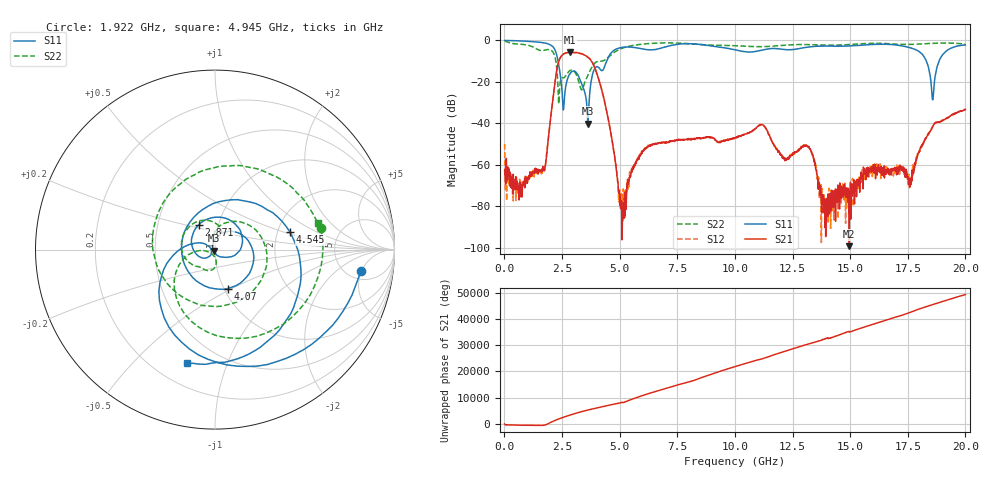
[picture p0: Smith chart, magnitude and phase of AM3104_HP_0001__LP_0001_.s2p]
!Created with skrf (http://scikit-rf.org).
# Hz S RI R 50.0
!freq ReS11 ImS11 ReS21 ImS21 ReS12 ImS12 ReS22 ImS22
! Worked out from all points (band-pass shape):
!   1601 points, 10 MHz to 20 GHz, reference 50 ohm
!   highest |S21| = -5.71 dB at 2.834 GHz (marker M1); lowest = -99.2 dB at 14.97 GHz (marker M2)
!   |S21| within 3 dB of the highest: 2.406 GHz to 3.696 GHz (1.29 GHz wide, 42.3 % of centre)
!   lowest |S11| = -40.1 dB at 3.621 GHz (marker M3), VSWR 1.02, Z = 49.2 - j0.591 ohm
!   |S11| at or under -10 dB: 2.33 GHz to 4.433 GHz (2.103 GHz wide, 62.2 % of centre); 18.31 GHz to 18.86 GHz (548.1 MHz wide, 2.95 % of centre)
!   |S22| runs from -30.6 to -0.2 dB; largest |S21 - S12| = 0.004
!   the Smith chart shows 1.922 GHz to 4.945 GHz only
!   S11 on the Smith chart (normalised r, x): 1.922 GHz: 6.62, -4.82; 2.871 GHz: 0.81, +0.23; 4.07 GHz: 1.05, -0.48; 4.545 GHz: 2.34, +0.56; 4.945 GHz: 0.33, -0.73
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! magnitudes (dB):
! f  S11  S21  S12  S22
! 10 MHz  0.0  -62.6  -50.0  -0.2
! 597.2 MHz  -0.2  -70.2  -72.1  -1.7
! 1.684 GHz  -1.1  -62.6  -62.4  -4.8
! 1.922 GHz  -1.7  -45.4  -45.7  -4.4
! 2.334 GHz  -10.2  -11.1  -11.1  -24.6
! 2.559 GHz  -33.5  -6.6  -6.6  -18.0
! 2.834 GHz  -16.2  -5.7  -5.7  -14.6
! 2.871 GHz  -15.6  -5.7  -5.7  -14.4
! 3.346 GHz  -20.9  -6.5  -6.5  -23.8
! 3.621 GHz  -40.1  -8.1  -8.0  -16.7
! 4.07 GHz  -12.8  -17.9  -17.9  -10.1
! 4.545 GHz  -7.4  -40.1  -40.2  -7.7
! 4.945 GHz  -3.7  -72.3  -72.1  -4.5
! 6.682 GHz  -4.0  -49.5  -49.6  -1.2
! 10.01 GHz  -4.5  -47.2  -47.0  -2.5
! 13.34 GHz  -2.9  -54.3  -54.7  -2.1
! 13.9 GHz  -2.7  -79.9  -80.2  -2.2
! 14.97 GHz  -2.6  -99.2  -73.2  -1.9
! 16.68 GHz  -1.8  -63.8  -63.2  -1.5
! 17.63 GHz  -3.6  -67.8  -67.0  -1.9
! 18.58 GHz  -28.6  -41.7  -41.5  -1.4
! 20 GHz  -2.2  -33.2  -33.3  -1.7
